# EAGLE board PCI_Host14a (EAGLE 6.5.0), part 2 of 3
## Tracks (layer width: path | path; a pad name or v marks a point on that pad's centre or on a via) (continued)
IDSEL2  (via drill 0.2, 0.3) (continued)
  Top 0.254: IC1.91 44.39,56.75 41.77,54.13 24.62,54.13 | v12.4,63.58 12.42,63.6 14.95,63.6 15.49,63.06 v15.88,63.06 15.8,63.06
  Top 0.305: v15.87,54.76 15.89,54.74 15.89,54.25 v17.05,53.09 | v20.35,49.96 v21.94,49.96 | v24.56,54.08 24.62,54.13
  Bottom 0.152: X1.J3-D18 6.1,64.21 11.76,64.21 v12.4,63.58
  Bottom 0.254: v12.4,63.58
  Bottom 0.305: 15.87,54.74 v15.88,63.06 | 15.87,54.74 15.87,54.6 | v17.05,53.09 17.05,50.44 17.53,49.96 v20.35,49.96 | v21.94,49.96 21.94,50.97 22.72,51.75 23.51,51.75 24.78,53.02 24.78,53.86 v24.56,54.08 | v15.87,54.76 15.87,54.74
IDSEL3  (via drill 0.2, 0.3)
  Top 0.152: v52.56,26.04 52.56,26.99 51.93,27.62 51.93,33.81 49.23,36.51 49.23,39.69 v48.91,40 | 45.57,45.24 45.56,45.23 v45.26,45.23 | 1.28,20.48 1.28,22.38
  Top 0.254: v47.96,45.24 45.57,45.24 | v44.78,47.15 44.78,47.62 v43.83,48.58 | IC1.90 44.1,57.26 41.76,54.92 v41.45,54.92 | v1.44,59.69 1.44,41.12 2.08,40.48 2.08,25.08 1.6,24.61 1.6,23.65 1.44,23.49 | 1.44,23.49 | 1.44,23.49 1.28,23.34 1.28,22.38 | 1.28,20.48 1.28,20 1.6,19.68 1.6,19.21 1.76,19.05 1.76,18.57 2.68,17.65
  Top 0.305: v17.54,25.2 17.54,18.34 16.93,17.73 v15.71,17.73 | v2.76,17.73 2.68,17.65
  Bottom 0.152: v43.83,48.58 43.83,48.89 | v45.26,45.23 45.26,46.67
  Bottom 0.254: 1.57,65.21 X1.J3-D19 | 1.57,65.21 | v41.45,54.92 41.45,51.28 43.83,48.89 | v48.91,40 48.91,44.13 v47.96,45.24 | 45.26,46.67 v44.78,47.15 | 1.57,65.21 | 1.57,65.21 1.28,64.93 1.28,59.85 v1.44,59.69
  Bottom 0.305: v17.54,25.2 18.76,26.42 52.14,26.42 52.44,26.11 v52.56,26.04 | v2.76,17.73 v15.71,17.73
INTA#  (via drill 0.2, 0.3)
  Top 0.152: 9.18,85.21 10.33,86.2 v12.71,86.2 | 64.17,80.06 64.17,71.37 64.33,71.22 64.33,70.61 64.48,70.46 64.48,70 64.94,69.53 64.94,67.76 v63.98,66.8 | v59.45,63.3 v59.45,59.59 | v64.31,56.61 v70.82,56.61 | IC1.47 64.05,62.76 64.2,62.9 v64.75,63.44
  Top 0.254: X1.J3-B29 9.18,85.21 | v15.33,86.12 17.87,86.12 18.75,85.25 22.4,85.25
  Top 0.305: v73.93,57.2 73.93,55.07 73.78,54.92 73.78,39.52 74.54,39.52 74.69,39.37 74.69,37.69 R2.2 | v25.77,92.41 25.77,86.46 23.94,86.46 23.79,86.31 23.64,86.31 23.48,86.16 23.48,86 23.33,85.85 23.33,85.24 22.42,85.24 22.4,85.25 | v62.35,98.35 62.35,99.42 62.5,99.57 63.87,99.57 63.87,98.5 63.72,98.35 63.72,88.9 63.87,88.75 64.33,88.75 64.33,85.85 64.17,85.7 64.17,84.02 64.33,83.87 64.33,80.21 64.17,80.06 | v25.41,93.98 v25.41,95.73 | v25.41,98.9 28.72,98.9 28.95,99.12 v29.3,99.12
  Bottom 0.152: v59.45,59.59 59.51,59.53 60.82,59.53 63.52,56.83 63.52,56.77 63.71,56.57 64.27,56.57 v64.31,56.61 | 59.76,66.95 63.83,66.95 v63.98,66.8 | 73.88,57.15 71.35,57.15 v70.82,56.61 | v59.45,63.3 63.79,63.3 64.15,63.66 64.53,63.66 v64.75,63.44
  Bottom 0.254: v12.71,86.2 15.02,86.2 v15.33,86.12
  Bottom 0.305: v62.35,98.35 62.19,98.2 34.06,98.2 33.19,99.06 29.36,99.06 v29.3,99.12 | 59.76,66.95 59.6,66.8 59.6,64.52 59.45,64.36 v59.45,63.3 | 73.88,57.15 v73.93,57.2 | v25.77,92.41 25.77,93.62 v25.41,93.98 | v25.41,95.73 v25.41,98.9 | 63.52,56.83
INTB#  (via drill 0.2, 0.3)
  Top 0.152: 7.12,85.21 v8.03,84.3 | 66.16,83.57 66.16,80.52 | IC1.48 63.44,63.26 63.99,63.82 64.47,64.29 | 64.47,64.29 | 64.47,64.29 64.63,64.45 64.63,64.93 v64.65,64.93 65,65.31 65,65.46 65.1,65.56 | 66.31,80.37 66.31,66.79 65.8,66.28 65.8,66.26 65.1,65.56 | 65.1,65.56 | 78.5,61.47 78.5,64.78 v78.35,64.94
  Top 0.254: X1.J3-C29 7.12,85.21 | 22.72,82.87 18.91,82.87 17.8,83.98 17.32,83.98 16.29,85.01 v14.46,85.01
  Top 0.305: v72.41,53.7 72.56,53.54 72.56,39.37 72.25,39.37 72.1,39.22 72.1,37.69 R2.3 | v78.2,53.7 78.35,53.85 78.35,59.49 78.2,59.64 78.2,61.32 78.35,61.47 78.5,61.47 | v23.18,82.35 23.18,82.8 22.72,82.8 22.72,82.87 | v27.6,82.35 31.41,82.35 v31.41,79.91 | v39.64,79.91 39.49,80.06 39.49,83.72 v39.64,83.87 | v66.31,83.72 66.16,83.57 | 66.16,80.52 66.31,80.37
  Bottom 0.152: 13.75,84.3 13.67,84.22 8.11,84.22 v8.03,84.3 | v78.35,64.94 64.82,64.94 v64.65,64.93
  Bottom 0.254: 13.75,84.3 v14.46,85.01
  Bottom 0.305: v72.41,53.7 72.56,53.54 78.04,53.54 v78.2,53.7 | v23.18,82.35 v27.6,82.35 | v31.41,79.91 v39.64,79.91 | v39.64,83.87 39.79,84.02 64.94,84.02 65.09,83.87 65.09,83.72 v66.31,83.72
INTC#  (via drill 0.2, 0.3)
  Top 0.152: 4.3,88.58 13.99,88.58 | v65.55,84.48 65.55,80.37 | 65.7,80.21 65.7,67.27 v64.94,66.52 64.57,66.14 64.41,66.14 63.99,65.72 63.99,64.51 63.24,63.76 IC1.49
  Top 0.254: v4.14,88.42 | v4.14,88.42 4.3,88.58 | 13.99,88.58 v14.62,87.95 | v17.32,85.25 | v17.32,85.25 17.8,84.77 18.11,84.77 18.59,84.3 | 18.59,84.3 | 18.59,84.3 18.75,84.14 21.92,84.14
  Top 0.305: v69.51,43.03 69.51,37.69 R2.4 | v75.15,43.03 75.3,43.18 75.3,48.36 75.15,48.51 75.15,57.51 v75,57.66 | v85.36,57.81 85.21,57.96 85.21,66.04 v85.36,66.19 | 26.23,84.78 26.23,85.85 24.09,85.85 23.94,85.7 23.94,84.18 21.96,84.18 21.92,84.14 | 26.23,84.78 26.07,84.63 | v32.17,82.42 32.17,77.01 31.68,76.52 28.59,76.52 28.11,76.99 | 65.55,80.37 65.7,80.21 | 26.23,84.78 26.22,84.78 26.05,84.61 26.05,78.74 25.73,78.42 25.73,78.11 26.21,77.63 27.48,77.63 28.11,76.99 | 28.11,76.99 | v38.12,84.78 38.12,82.89 v37.64,82.42
  Bottom 0.152: 5.09,85.41 3.98,86.52 3.98,88.27 | 79.87,66.95 79.85,66.93 67.26,66.93 66.85,66.52 v64.94,66.52
  Bottom 0.254: X1.J3-D29 5.09,85.41 | 3.98,88.27 v4.14,88.42 | v14.62,87.95 14.46,88.11 17.16,85.41 | 17.16,85.41 | 17.16,85.41 v17.32,85.25
  Bottom 0.305: v69.51,43.03 69.66,43.18 75,43.18 v75.15,43.03 | v75,57.66 75.15,57.81 75.3,57.81 75.45,57.96 85.21,57.96 v85.36,57.81 | v85.36,66.19 80.94,66.19 80.79,66.34 80.79,66.95 79.87,66.95 | v38.12,84.78 38.12,84.48 39.18,84.48 39.33,84.63 65.39,84.63 v65.55,84.48 | v32.17,82.42 v37.64,82.42
INTD#  (via drill 0.2)
  Top 0.152: X1.J3-B28 9.33,83.21 10.33,84.22 15.81,84.22 | v74.54,79.15 73.17,79.15 v73.17,80.67 | v63.57,80.52 63.57,71.22 63.72,71.07 63.72,70.46 63.87,70.31 63.87,69.55 64.02,69.39 64.17,69.39 64.17,68.61 63.36,67.79 63.36,64.93 63.04,64.61 62.5,64.61 IC1.50
  Top 0.254: 15.81,84.22 15.93,84.09
  Top 0.305: v67.38,43.79 67.53,43.64 67.53,39.52 67.22,39.52 67.07,39.37 67.07,37.69 R2.5 | v96.03,47.3 v96.03,43.79 | v92.22,54.92 92.06,55.07 92.06,58.11 92.22,58.27 92.22,59.18 92.06,59.33 91.15,59.33 91.15,61.92 91,62.08 91,62.38 90.84,62.53 89.02,62.53 89.02,70.92 v89.17,71.07 | v16.02,84.33 16.02,84.18 15.93,84.09 | v18.76,91.19 18.46,91.19 18.46,91.49 18.3,91.64 18.15,91.64 v18.15,95.3 | v54.42,113.59 54.42,112.52 54.57,112.37 54.57,111.76 54.42,111.61 54.42,110.08 54.57,109.93 54.57,109.17 54.73,109.02 54.88,109.02 54.88,104.75 55.03,104.6 57.62,104.6 57.62,97.89 57.47,97.74 57.47,88.44 57.62,88.29 58.23,88.29 58.23,80.82 v58.08,80.67 | v11.45,98.2 12.94,98.2 13.19,97.95 13.19,95.3 v13.35,95.14
  Bottom 0.152: 66.16,80.82 71.95,80.82 | 63.72,80.67 66,80.67 | v58.08,80.67 63.57,80.67
  Bottom 0.305: v67.38,43.79 78.35,43.79 78.5,43.94 78.5,44.09 89.47,44.09 89.63,43.94 89.63,43.79 v96.03,43.79 | v96.03,47.3 96.03,47.6 95.72,47.6 95.57,47.75 95.57,50.19 95.72,50.34 95.88,50.34 96.03,50.5 96.03,51.56 98.62,51.56 98.77,51.71 98.77,53.24 98.92,53.39 98.92,54.76 97.25,54.76 97.09,54.92 v92.22,54.92 | v89.17,71.07 89.02,71.22 85.21,71.22 85.05,71.07 84.14,71.07 83.99,71.22 83.99,79.15 v74.54,79.15 | v73.17,80.67 72.1,80.67 71.95,80.82 | 66,80.67 66.16,80.82 | 63.72,80.67 v63.57,80.52 63.57,80.67 | v16.02,84.33 16.17,84.48 17.85,84.48 18,84.63 18,84.78 18.15,84.94 18.15,86.31 17.54,86.31 17.39,86.46 17.39,89.05 17.54,89.2 18.76,89.2 18.91,89.36 18.91,91.19 v18.76,91.19 | v11.45,98.2 11.29,98.35 11.29,106.84 12.09,107.64 18.3,107.64 19.07,108.41 19.07,112.94 19.87,113.74 54.27,113.74 v54.42,113.59 | v18.15,95.3 13.51,95.3 v13.35,95.14
IRDY#  (via drill 0.2, 0.3)
  Top 0.152: IC1.55 58.15,65.33 58.32,65.17 60.86,65.17 v60.98,65.28 | X1.J3-C13 7.03,53.21 6.05,52.23 5.69,52.23 5.67,52.21 4.42,52.21 4.38,52.17 4.16,52.17 v4.14,52.19 | v7.04,25.06 12.7,25.06
  Top 0.254: 12.7,25.06 12.89,25.06 v13.51,24.45
  Top 0.305: v13.51,29.53 21.92,29.53 22.72,30.32 37.16,30.32 37.2,30.38 v37.2,28.09 | v77.74,64.21 77.74,59.33 77.89,59.18 77.89,54.3 77.59,54 v77.59,52.93 | v74.39,52.93 74.23,52.78 74.23,40.59 75.15,39.67 75.15,39.22 75.61,38.76 75.61,35.56 74.23,34.19 74.23,32.21 73.32,31.29 v73.32,30.53 | v76.83,30.23 76.83,29.31 76.98,29.16 v76.98,17.27 | v55.64,16.66 55.64,17.42 55.49,17.58 v55.49,20.17 | v43.45,20.32 43.6,20.47 43.6,27.94 v43.45,28.09
  Bottom 0.152: 82.16,65.13 80.94,65.13 80.94,64.68 80.47,64.21 v77.74,64.21 67.8,64.21 | v4.14,52.19 3.21,52.19 2.69,51.67 2.69,50.76 2.34,50.4 2.16,50.4 1.92,50.17 1.92,41.12 2.71,40.32 2.71,38.38 2.91,38.18 2.91,27.58 3.35,27.15 3.51,27.15 4.62,26.04 6.07,26.04 v7.04,25.06 | v13.51,24.45 v13.51,29.53
  Bottom 0.305: v60.98,65.28 60.98,64.21 67.8,64.21 68.29,64.21 | 82.16,65.13 R1.3 | v77.59,52.93 77.43,53.09 74.54,53.09 v74.39,52.93 | v73.32,30.53 73.62,30.23 v76.83,30.23 | v76.98,17.27 76.83,17.42 62.19,17.42 62.04,17.27 61.13,17.27 60.52,16.66 v55.64,16.66 | v55.49,20.17 55.34,20.02 44.67,20.02 44.36,20.32 v43.45,20.32 | v43.45,28.09 43.3,27.94 37.35,27.94 v37.2,28.09
LED_A  (via drill 0.2, 0.3)
  Top 0.152: v63.41,68.94 63.26,69.09 63.26,70.16 63.11,70.31 63.11,70.92 62.96,71.07 62.96,80.06 | 46.19,64.36 46.19,65.27 45.89,65.56 45.89,67.41 v46.03,67.55 | v74.15,98.42 74.15,99.7
  Top 0.305: 62.96,80.06 62.8,80.21 62.65,80.21 62.65,86.16 62.8,86.31 62.96,86.31 62.96,88.75 63.11,88.9 v63.11,98.81 | 74.15,99.7 R5.1 | IC1.76 46.19,64.36
  Bottom 0.152: 71.71,98.96 73.62,98.96 v74.15,98.42 | v63.41,68.94 63.29,69.22 61.29,69.22 60.98,68.9 59.86,68.9 59.07,69.69 57.64,69.69 57.32,70.01 51.77,70.01 51.13,69.37 51.13,67.63 50.66,67.15 46.53,67.15 46.13,67.55 v46.03,67.55
  Bottom 0.254: 71.61,98.96 71.71,98.96
  Bottom 0.305: v63.11,98.81 63.26,98.96 71.61,98.96
LED_B  (via drill 0.2)
  Top 0.152: v71.76,77.76 71.76,69.42 v72.08,69.1
  Top 0.305: v91,67.41 91,66.34 90.84,66.19 90.24,66.19 90.24,65.13 LED2.C | v46.95,68.17 46.95,67.72 47.26,67.72 47.41,67.56 47.41,66.34 48.02,66.34 IC1.75 | v47.56,74.57 v47.56,78.38
  Bottom 0.152: 71.03,78.23 71.03,78.21 71.29,77.95 71.58,77.95 v71.76,77.76 | v72.08,69.1 72.08,69.06 72.56,68.58 80.43,68.58 80.79,69.09
  Bottom 0.305: 80.79,69.09 84.29,69.09 84.45,68.94 84.45,67.56 89.78,67.56 89.93,67.72 90.84,67.72 91,67.56 v91,67.41 | v46.95,68.17 46.95,69.09 46.8,69.24 46.65,69.24 46.65,73.36 46.5,73.36 46.34,73.51 46.34,74.57 v47.56,74.57 | v47.56,78.38 47.72,78.23 57.77,78.23 57.93,78.38 70.88,78.38 71.03,78.23
LOCK#  (via drill 0.2, 0.3)
  Top 0.152: 12.71,50.64 14.86,50.64 17.16,48.34 17.32,48.34 18.35,47.31 | 18.35,47.31 | 18.35,47.31 18.43,47.23 24.14,47.23 24.22,47.15 26.53,47.15 v27,47.62 | v27,47.62
  Top 0.305: v12.56,50.64 12.66,50.65 12.71,50.64 | v40.18,87.95 40.34,87.79 40.34,83.33 v40.4,83.26 40.5,83.17 40.5,79.38 39.23,78.11 35.89,78.11 v31.29,73.5
  Bottom 0.152: 7.95,50.17 12.08,50.17 | 72.73,82.22 73.83,81.12 73.83,77.15 73.99,76.99 73.99,74.93 75.1,73.82 75.1,72.87 75.26,72.71 R1.6 | 58.69,81.89 65.7,81.89 65.85,82.04 71.95,82.04 | 31.29,72.39 29.86,70.96 29.86,68.74 29.54,68.42 29.54,57.47 27.96,55.88 27.96,48.58 v27,47.62
  Bottom 0.254: X1.J3-C11 7.09,49.31 7.95,50.17 | 12.08,50.17 v12.56,50.64
  Bottom 0.305: v40.4,83.26 40.55,83.41 55.03,83.41 55.18,83.26 55.18,82.04 58.54,82.04 58.69,81.89 | 71.95,82.04 72.1,82.19 72.71,82.19 72.73,82.22 | 39.54,88.27 v30.81,88.27 | 39.54,88.27 | 39.54,88.27 39.86,88.27 v40.18,87.95 | 31.29,72.39 v31.29,73.5
N$2  (via drill 0.2)
  Top 0.305: v92.22,93.93 92.22,88.14 92.37,87.99 92.37,70.46 92.06,70.46 91.91,70.31 91.91,70 91.76,69.85 91.76,67.26 92.83,67.26 92.98,67.11 92.98,65.13 LED2.A
  Bottom 0.254: 86.46,93.78 86.46,99.93
  Bottom 0.305: v92.22,93.93 92.06,93.78 86.46,93.78 | R5.2 85.11,101.28 86.46,99.93
N$3
  Top 0.305: J2.4 20.28,112.22 17.85,112.22 J2.2 | 37.05,112.22 35.68,112.22 J3.2 | 37.05,112.22 38.12,112.22 J3.4 | 37.05,112.22 37.05,108.1 36.44,108.1 36.29,107.95 36.29,103.23 JP3.1
  Bottom 0.305: J2.4 20.44,112.06 21.2,112.06 22.27,111 23.33,111 24.4,112.06 35.52,112.06 J3.2
N$4  (via drill 0.2)
  Top 0.152: 76.37,48.82 v76.37,102.31
  Top 0.305: v84.6,16.05 84.6,21.39 L1.2 | 66.08,14.45 66.16,14.38 66.92,14.38 66.92,12.7 C18.+ 66.92,12.55 | 66.08,14.45 66,14.53 66,18.34 IC3.4 | 73.47,19.86 69.36,19.86 69.2,20.02 69.2,25.65 IC3.20 | 76.37,48.82 76.52,48.67 76.52,39.22 76.37,39.06 76.06,39.06 76.06,34.04 75.91,33.88 74.69,33.88 74.69,29.16 74.84,29.01 74.84,21.84 74.69,21.69 73.47,21.69 73.47,19.86 | v66.16,14.83 66.16,14.53 66.08,14.45 | R9.2 70.88,3.56 70.88,7.52 R8.2 70.88,7.67 v70.88,14.83 | v73.47,15.75 73.47,19.86
  Bottom 0.305: v84.6,16.05 81.85,16.05 81.7,16.2 76.22,16.2 76.06,16.05 76.06,15.75 74.39,15.75 74.31,15.67 | 74.31,15.67 74.23,15.6 74.23,14.83 v70.88,14.83 v66.16,14.83 59.76,14.83 JP5.1 | v76.37,102.31 76.22,102.46 69.2,102.46 69.2,102.16 69.05,102.01 67.07,102.01 67.07,102.92 66.92,103.07 65.85,103.07 C17.1 | v73.47,15.75 74.23,15.75 74.31,15.67
N$5
  Top 0.305: LED3.A 83.53,4.01 82.31,4.01 82.31,5.38 82.16,5.54 81.79,5.54 81.3,6.03 81.3,7.3 R8.1
N$9
  Bottom 0.305: IC2.1 78.96,41.5 79.87,41.5 80.03,41.35 80.03,36.47 86.58,36.47 C11.1
N$10  (via drill 0.2)
  Top 0.305: 16.62,107.04 12.82,107.04 12.82,102.46 JP9.1 | 16.62,107.04 17.22,107.04 17.8,107.61 | v66.31,87.22 66.46,87.38 66.46,91.95 66.31,92.1 66.31,92.86 66.46,92.86 66.61,93.02 66.61,95.61 66.77,95.76 66.77,96.67 66.61,96.83 66.61,96.98 66.46,96.98 66.31,97.13 66.31,100.64 66.46,100.79 66.46,101.7 66.16,101.7 66,101.85 65.39,101.85 65.24,101.7 63.72,101.7 63.57,101.85 63.57,109.02 63.72,109.17 63.72,114.35 56.4,114.35 56.25,114.2 56.25,113.74 v56.1,113.59 56.1,113.62 55.42,114.3 53.2,114.3 53.04,114.14 16.84,114.14 15.73,113.03 15.73,110.81 16.69,109.85 16.62,109.78 16.62,107.04 | v105.32,86.77 105.48,86.61 105.48,64.36 104.87,63.75 104.71,63.75 104.71,63.6 104.56,63.45 104.56,61.62 104.71,61.47 104.87,61.47 104.87,48.36 v104.71,48.21 | v97.4,47.3 97.55,47.14 97.55,44.55 v97.4,44.4 | v77.89,44.55 77.74,44.4 77.74,39.22 77.89,39.06 78.5,39.06 78.5,36.17 78.35,36.02 77.74,36.02 77.74,32.21 77.59,32.05 77.43,32.05 77.43,31.29 77.59,31.14 77.59,29.31 77.43,29.16 77.43,21.84 77.59,21.69 78.81,21.69 78.81,21.39 78.96,21.23 78.96,20.78 79.11,20.62 79.11,20.02 78.96,19.86 v78.96,18.19 | X3.2 29.43,7.67 29.43,16.66 C26.+ 29.43,16.81 v29.43,19.56 | v15.71,21.84 16.93,20.62 v16.93,19.86
  Bottom 0.305: v105.32,86.77 94.2,86.77 94.05,86.61 82.77,86.61 82.77,87.38 82.62,87.53 75.16,87.53 74.79,87.15 72.88,87.15 72.72,87.31 66.4,87.31 v66.31,87.22 | v104.71,48.21 101.97,48.21 101.82,48.06 101.82,47.9 101.51,47.9 101.36,47.75 101.36,47.45 101.06,47.45 100.9,47.3 v97.4,47.3 | v97.4,44.4 97.25,44.55 94.81,44.55 94.66,44.4 89.93,44.4 89.63,44.7 78.04,44.7 v77.89,44.55 | v78.96,18.19 78.81,18.34 61.59,18.34 61.43,18.19 59.76,18.19 JP10.3 59.6,18.19 58.84,18.19 57.62,19.41 55.49,19.41 55.34,19.56 44.06,19.56 v44.06,19.71 43.91,19.56 39.49,19.56 39.33,19.41 32.93,19.41 32.78,19.56 30.95,19.56 30.8,19.41 29.43,19.41 v29.43,19.56 29.28,19.41 24.55,19.41 24.4,19.56 22.57,19.56 22.27,19.86 v16.93,19.86 | v15.71,21.84 14.34,21.84 JP11.1
N$11
  Top 0.305: C11.2 89.17,36.63 89.17,38.3 89.02,38.46 87.64,38.46 87.64,43.03 87.49,43.18 83.99,43.18 83.99,41.5 IC2.3
N$13
  Top 0.305: IC2.4 86.58,41.35 86.58,38 86.73,37.85 88.1,37.85 88.1,36.17 88.25,36.02 88.25,33.12 88.41,32.97 89.02,32.97 89.02,32.66 89.17,32.51 89.17,30.38 89.32,30.23 91.91,30.23 91.91,34.65 92.06,34.8 92.52,34.8 92.52,36.47 C12.1
N$14
  Top 0.305: J1.2 53.36,112.06 53.36,111.15 53.2,111 48.94,111 48.94,103.23 JP1.1
N$15  (via drill 0.2)
  Top 0.152: 75.76,99.26 75.76,76.1 75.61,75.95 74.84,75.95 74.84,70.46 75,70.31 75.76,70.31 75.76,48.67
  Top 0.305: v22.88,100.48 22.88,100.18 20.74,100.18 20.59,100.33 20.59,103.53 20.44,103.53 20.28,103.68 20.28,109.47 J2.3 | 75.76,99.26 v75.61,99.42 | 75.76,48.67 75.91,48.51 75.91,39.83 v75.76,39.67
  Bottom 0.305: v22.88,100.48 23.03,100.64 29.08,100.64 29.99,99.72 34.15,99.72 34.3,99.87 39.49,99.87 39.64,99.72 46.8,99.72 46.95,99.87 46.95,100.03 54.88,100.03 55.03,99.87 55.03,99.72 60.98,99.72 61.13,99.57 74.39,99.57 74.54,99.42 v75.61,99.42 | v75.76,39.67 75.76,34.19 70.27,34.19 70.12,34.04 59.3,34.04 59.15,34.19 59.15,34.34 58.08,34.34 57.93,34.19 57.93,33.43 56.71,33.43 56.55,33.27 56.4,33.27 56.25,33.12 56.25,32.97 54.42,32.97 54.27,32.82 54.27,31.29 53.2,31.29 JP2.8 53.05,31.29 52.14,31.29 52.14,30.38 51.98,30.23 51.22,30.23 51.07,30.07 50.16,30.07 50,30.23 49.55,30.23 49.39,30.38 49.09,30.38 49.09,31.14 48.94,31.29 48.17,31.29 JP2.4
N$16
  Top 0.305: C12.2 95.11,36.63 95.11,39.52 94.96,39.67 92.67,39.67 92.67,42.72 92.52,42.88 92.37,42.88 92.37,43.03 92.22,43.18 89.02,43.18 89.02,41.5 IC2.5
N$17  (via drill 0.2)
  Top 0.305: v81.09,32.51 80.94,32.66 80.94,39.98 81.09,40.13 81.4,40.13 81.4,41.35 IC2.2
  Bottom 0.305: v81.09,32.51 79.87,32.51 79.87,31.75 79.72,31.6 78.65,31.6 C13.2
N$18  (via drill 0.2)
  Top 0.305: v93.74,56.44 93.74,50.95 94.05,50.95 94.2,50.8 94.2,49.12 IC2.10
  Bottom 0.305: v93.74,56.44 89.47,56.44 JP4.2
N$19
  Bottom 0.305: IC2.9 96.79,49.12 99.38,49.12 99.53,49.28 99.53,49.58 100.9,49.58 101.06,49.73 101.06,50.19 101.21,50.19 101.36,50.34 101.36,50.5 101.67,50.5 101.82,50.65 101.82,54.15 104.71,54.15 104.87,54.3 104.87,55.83 105.32,55.83 105.48,55.98 105.48,61.47 98.01,61.47 97.86,61.32 97.86,60.25 97.25,60.25 97.09,60.1 93.13,60.1 92.98,59.94 92.98,57.81 91.15,57.81 91,57.96 88.56,57.96 88.41,57.81 88.41,57.2 88.25,57.05 88.25,55.98 88.41,55.83 88.41,54 89.32,54 JP4.4
N$21
  Top 0.305: C10.1 90.24,31.6 90.24,34.95 90.39,35.1 91.15,35.1 91.15,39.52 91.3,39.67 91.61,39.67 91.61,41.35 IC2.6
N$22  (via drill 0.2)
  Top 0.305: JP7.5 90.39,78.38 90.39,77.47 91.61,76.25 91.61,75.49 90.39,74.27 90.39,73.36 JP7.1 | v82.62,56.74 82.62,54.92 82.46,54.76 82.46,53.7 82.62,53.7 82.77,53.54 82.77,51.56 83.83,51.56 83.99,51.41 83.99,49.12 IC2.14 | v84.75,56.74 84.6,56.9 84.6,66.5 84.75,66.65 84.75,69.09 84.6,69.24 84.6,71.68 v84.75,71.83
  Bottom 0.305: v82.62,56.74 v84.75,56.74 | v84.75,71.83 89.17,71.83 89.32,71.98 89.32,73.36 90.24,73.36 JP7.1
N$23
  Top 0.305: 89.4,77.7 90.39,76.71 90.39,75.95 JP7.3 | 89.4,77.7 89.17,77.93 89.17,78.84 90.39,80.06 90.39,80.82 JP7.7 | IC2.13 86.58,49.12 86.58,52.32 86.73,52.48 87.8,52.48 87.8,52.78 87.95,52.93 87.95,53.39 88.1,53.54 88.1,54.3 87.95,54.46 87.95,55.98 88.1,56.13 88.1,57.05 88.25,57.2 88.41,57.2 88.41,72.29 88.56,72.44 88.86,72.44 88.86,72.75 89.02,72.9 89.02,73.81 89.17,73.97 89.32,73.97 89.32,77.62 89.4,77.7
N$24
  Top 0.305: JP7.8 87.8,80.82 87.8,80.06 86.58,78.84 86.58,75.49 87.8,74.27 87.8,73.36 JP7.2
  Bottom 0.305: J6.2 100.29,81.43 98.47,81.43 98.47,79.3 98.31,79.15 97.86,79.15 97.7,78.99 97.55,78.99 97.55,78.84 97.4,78.69 96.03,78.69 J4.3 95.88,78.69 92.06,78.69 91.91,78.84 91.91,79.3 91.61,79.3 91.45,79.45 91,79.45 90.84,79.6 89.93,79.6 89.78,79.76 89.78,79.91 89.02,79.91 88.86,80.06 88.86,80.98 87.95,80.98 JP7.8
N$26
  Top 0.305: JP7.6 87.8,78.38 87.8,75.95 JP7.4
  Bottom 0.305: J6.3 100.29,78.69 98.62,78.69 98.47,78.54 98.01,78.54 97.86,78.38 97.86,76.4 97.7,76.25 96.03,76.25 J4.2 95.88,76.25 94.2,76.25 94.2,76.71 94.05,76.86 91,76.86 90.84,77.01 89.78,77.01 89.63,76.86 89.32,76.86 89.17,76.71 88.86,76.71 88.86,76.1 88.71,75.95 87.95,75.95 JP7.4
N$27  (via drill 0.2)
  Top 0.305: IC2.7 94.2,41.5 v94.2,45.77 93.28,45.77 93.13,45.92 93.13,55.52 v92.98,55.68
  Bottom 0.305: v94.2,45.77 100.29,45.77 J7.3 | v92.98,55.68 94.35,55.68 94.35,55.98 94.5,56.13 95.88,56.13 J5.2
N$28  (via drill 0.2)
  Top 0.305: v98.92,41.5 98.77,41.66 98.77,47.14 98.85,47.22 | 98.85,47.22 98.92,47.3 100.29,47.3 100.29,48.36 J7.2 | J5.3 95.88,58.72 95.88,57.81 96.03,57.66 98.31,57.66 98.31,54.61 98.77,54.15 98.77,47.3 98.85,47.22
  Bottom 0.305: v98.92,41.5 96.79,41.5 IC2.8
N$33  (via drill 0.2)
  Top 0.305: v92.98,88.44 92.98,68.94 LED1.A
  Bottom 0.305: v92.98,88.44 84.29,88.44 R4.2
N$35  (via drill 0.2)
  Top 0.305: v71.64,28.55 71.8,28.4 71.8,25.81 IC3.16 | v87.03,28.55 87.03,25.96 C15.1 | v97.4,24.43 97.4,23.37 97.55,23.22 97.55,19.41 98.31,19.41 98.47,19.56 100.14,19.56 X2.D-
  Bottom 0.305: v71.64,28.55 71.8,28.4 73.32,28.4 73.47,28.24 80.03,28.24 80.18,28.4 86.88,28.4 v87.03,28.55 | v97.4,24.43 97.25,24.28 95.42,24.28 95.27,24.13 90.24,24.13 90.08,24.28 87.95,24.28 87.8,24.43 87.8,25.81 87.03,25.81 C15.1
N$36  (via drill 0.2)
  Top 0.305: 21.88,19.33 21.05,18.49 21.05,16.81 C27.+ 21.05,16.66 v21.05,7.67 | 21.88,19.33 21.96,19.41 21.96,22.15 JP8.1 | 21.88,19.33 v21.96,19.25
  Bottom 0.305: JP6.1 16.47,15.75 18.3,15.75 19.22,16.66 20.89,16.66 C27.+ | v21.96,19.25 22.11,19.1 24.09,19.1 24.25,18.95 31.11,18.95 31.26,19.1 32.48,19.1 32.63,18.95 39.64,18.95 39.79,19.1 55.03,19.1 55.95,18.19 57.01,18.19 JP10.1 | v21.05,7.67 24.25,7.67 X3.1
N$37  (via drill 0.2)
  Top 0.305: v71.19,21.69 71.19,25.65 IC3.17 | v93.28,21.54 93.28,25.65 C19.1
  Bottom 0.305: v71.19,21.69 82.62,21.69 82.77,21.54 82.77,21.39 83.53,21.39 83.83,21.69 89.02,21.69 89.17,21.54 90.08,21.54 90.24,21.69 93.13,21.69 v93.28,21.54
N$38  (via drill 0.2)
  Top 0.305: v65.85,46.38 65.85,27.79 67.68,27.79 67.83,27.63 67.83,26.72 67.98,26.57 67.98,25.81 IC3.22 | v90.54,46.38 90.54,51.26 90.69,51.41 90.84,51.41 90.84,58.11 90.69,58.27 89.93,58.27 89.93,60.86 LED4.C
  Bottom 0.305: v65.85,46.38 71.49,46.38 71.64,46.53 90.39,46.53 v90.54,46.38
N$39  (via drill 0.2)
  Top 0.305: v67.38,19.71 67.38,25.65 IC3.23 | v83.38,18.95 83.38,14.99 83.53,14.83 83.53,14.07 83.38,13.92 83.38,6.76 83.53,6.76 LED3.C
  Bottom 0.305: v67.38,19.71 67.38,18.95 v83.38,18.95
N$40  (via drill 0.2)
  Top 0.305: v85.66,12.24 86.27,12.24 86.43,12.39 86.43,13.16 86.58,13.31 86.58,21.39 L1.1 86.58,21.54 v86.58,23.67 | v98.16,23.67 98.16,21.08 98.31,20.93 98.47,20.93 98.47,20.78 98.92,20.32 X2.D+
  Bottom 0.305: v85.66,12.24 78.2,12.24 C14.2 | v98.16,23.67 95.57,23.67 95.42,23.52 90.08,23.52 89.93,23.67 87.64,23.67 87.49,23.52 86.73,23.52 v86.58,23.67
N$41  (via drill 0.2)
  Top 0.152: 80.48,11.59 80.48,11.94
  Top 0.305: v92.67,62.84 92.67,61.01 LED4.A | v106.54,62.84 106.7,62.69 106.7,46.38 106.54,46.23 106.24,46.23 105.78,45.77 105.78,45.16 106.24,44.7 107.31,44.7 107.31,27.18 107.15,27.03 v106.54,27.03 | v81.55,26.87 81.55,26.42 81.7,26.26 81.7,25.2 81.55,25.04 81.55,17.27 81.4,17.12 80.48,17.12 80.48,11.94 | v79.57,3.56 79.57,8.74 80.48,9.65 80.48,11.59 80.48,11.79
  Bottom 0.305: v106.54,62.84 v92.67,62.84 | v106.54,27.03 94.81,27.03 94.66,27.18 81.7,27.18 81.55,27.03 v81.55,26.87 | v79.57,3.56 80.94,3.56 R9.1
N$46  (via drill 0.2)
  Top 0.305: v73.02,24.43 73.02,24.59 72.71,24.59 72.56,24.74 72.56,25.65 IC3.15 | v96.79,22.15 96.94,22 96.94,18.8 100.14,18.8 X2.VBUS | v83.22,22.15 83.22,25.65 C16.2
  Bottom 0.305: v73.02,24.43 75,24.43 75.15,24.28 82.16,24.28 82.31,24.43 82.31,25.65 83.07,25.65 C16.2 | v96.79,22.15 95.57,22.15 95.42,22.3 90.08,22.3 89.93,22.15 89.32,22.15 89.17,22.3 83.38,22.3 v83.22,22.15
N$101  (via drill 0.2)
  Top 0.305: v18.3,106.12 18.3,108.1 18,108.1 17.85,108.26 17.85,109.47 J2.1 | v69.36,106.73 69.51,106.58 69.51,94.54 v69.36,94.39 | v82.92,94.39 82.92,85.7 83.07,85.55 83.53,85.55 v83.53,85.39 | v104.26,85.24 104.41,85.09 104.41,69.55 v104.26,69.39 | v99.38,64.06 99.23,63.91 99.23,60.55 v99.38,60.4 | v103.65,55.07 103.8,54.92 103.8,51.11 v103.65,50.95 | v96.79,46.69 96.79,43.94 96.94,43.79 97.7,43.79 97.7,36.32 97.86,36.17 97.86,29.92 v97.7,29.77 | v54.27,30.23 54.27,31.75 54.12,31.9 54.12,32.05 53.97,32.21 53.81,32.21 53.66,32.36 53.2,32.36 53.05,32.51 53.05,32.66 v52.74,32.66
  Bottom 0.305: 48.55,32.44 48.48,32.51 47.72,32.51 47.56,32.36 47.11,32.36 46.95,32.21 46.65,32.21 46.65,31.45 46.5,31.29 45.58,31.29 JP2.2 | 48.55,32.44 48.63,32.36 49.39,32.36 49.55,32.21 49.55,31.45 49.7,31.29 50.61,31.29 JP2.6 | J2.1 17.69,109.47 | v18.3,106.12 18.46,105.97 28.82,105.97 28.97,106.12 30.8,106.12 30.95,106.27 52.59,106.27 52.74,106.43 52.74,106.58 52.9,106.58 53.05,106.73 53.81,106.73 53.97,106.88 69.2,106.88 v69.36,106.73 | v82.92,94.39 v69.36,94.39 | v83.53,85.39 83.68,85.55 94.5,85.55 94.66,85.7 104.1,85.7 104.26,85.55 v104.26,85.24 | v104.26,69.39 100.45,69.39 100.29,69.24 100.29,68.94 98.92,68.94 98.77,68.78 98.77,64.06 v99.38,64.06 | v99.38,60.4 99.38,60.1 99.08,60.1 98.92,59.94 98.92,59.64 98.77,59.49 98.77,56.74 98.92,56.59 99.08,56.59 99.23,56.44 99.23,56.29 99.38,56.13 99.53,56.13 99.69,55.98 99.69,55.83 99.84,55.68 99.84,55.07 v103.65,55.07 | v103.65,50.95 103.8,50.8 105.17,50.8 105.32,50.65 105.32,45.92 102.43,45.92 102.28,46.08 101.51,46.08 101.36,46.23 101.36,46.69 100.9,46.69 100.75,46.84 97.86,46.84 97.7,46.69 v96.79,46.69 | v97.7,29.77 86.43,29.77 86.27,29.62 86.12,29.62 85.97,29.46 78.65,29.46 78.5,29.62 76.52,29.62 76.37,29.77 63.87,29.77 63.72,29.92 62.96,29.92 62.8,30.07 62.8,30.23 62.5,30.23 62.35,30.38 62.35,30.68 62.19,30.84 62.19,31.6 62.04,31.75 61.89,31.75 61.74,31.9 61.74,32.21 61.43,32.21 61.28,32.36 57.77,32.36 57.62,32.21 57.47,32.21 57.32,32.05 57.32,31.9 57.16,31.75 57.16,30.99 57.01,30.84 56.86,30.84 56.71,30.68 56.71,30.23 56.25,30.23 56.1,30.07 55.34,30.07 55.18,30.23 v54.27,30.23
  Bottom 0.305: v52.74,32.66 52.59,32.82 48.78,32.82 48.63,32.66 48.63,32.51 48.55,32.44
PAR  (via drill 0.3)
  Top 0.152: 2.79,74.06 2.79,81.2 3.35,81.76 | X1.J3-D9 3.86,45.21 2.56,46.51 2.56,50.96 2.71,51.12 2.71,61.44 | 56.53,74.79 56.53,72.07 56.69,71.91 56.69,70.64 57.01,70.33 57.01,68.1 56.69,67.79 | 56.69,67.79 | 56.69,67.79 56.65,67.75 IC1.58 | 3.35,81.76 | 31.61,95.09
  Top 0.254: 2.71,73.98 2.79,74.06 | 2.71,73.98 | 2.71,73.98 2.48,73.74 2.48,71.83 2.79,71.52 2.79,67.07 3.19,66.67 3.19,64.37 3.83,63.74 3.83,63.02 3.35,62.55 3.35,62.07 2.71,61.44 | 3.35,81.76 3.35,89.06 | v15.41,94.3 15.26,94.14
  Top 0.305: 3.35,89.06 3.67,89.38 3.83,89.38 3.98,89.53 v3.98,89.69 4.84,90.55 10.2,90.55 10.41,90.77 12.04,90.77 12.28,91 12.28,93.48 13.11,94.32 15.39,94.32 v15.41,94.3 15.41,95.57 17,97.16 17.64,97.16 17.8,97.31 29.38,97.31 31.61,95.09 32.08,94.62 39.54,94.62 40.34,95.41 54.71,95.41 55.03,95.09 55.03,88.14 54.88,87.99 54.88,86.77 55.64,86.77 55.79,86.61 55.79,86.31 56.55,86.31 56.71,86.16 56.71,74.97 56.53,74.79
PERR#  (via drill 0.2, 0.3)
  Top 0.152: X1.J3-B10 9.6,47.21 10.49,48.1 | 10.49,48.1 10.57,48.18 12,48.18 12.71,47.47 | 10.49,48.1 | v74.54,77.78 73.02,77.78 73.02,74.88 | 12.71,47.47 | 12.71,47.47 12.79,47.39 15.18,47.39 16.37,46.2 16.84,46.2 16.92,46.2 17.56,45.56 29.07,45.56 29.23,45.72 29.7,45.72 v29.78,45.8 | IC1.43 67.6,60.76 68.44,61.59 68.44,63.5 67.33,64.61 67.33,64.93 68.59,66.2 68.59,70.48 69.23,71.12 69.23,74.31 v69.35,74.43
  Top 0.305: v73.17,74.73 73.02,74.88 | v41.3,75.15 39.96,75.15 39.54,75.56 37.64,75.56 37.32,75.25 v34.94,75.25
  Bottom 0.152: v29.78,45.8 29.78,47.39 29.86,47.47 | 29.86,47.47 | 29.86,47.47 30.02,47.62 30.02,54.93 31.45,56.36 | 31.45,60.64 32.88,62.07 32.88,64.29 33.35,64.77 | 58.08,75.95 68.69,75.95 69.07,75.56 69.07,74.7 v69.35,74.43 69.36,74.43 69.71,74.77 73.12,74.77 v73.17,74.73
  Bottom 0.305: v74.54,77.78 82.16,77.78 R1.8 | 58.08,75.95 57.93,76.1 42.24,76.1 v41.3,75.15 | 31.45,56.36 31.45,60.64 | v34.94,75.25 33.35,73.66 33.35,64.77
PME#  (via drill 0.3)
  Top 0.152: X1.J3-D10 5.47,47.21 6.44,48.18 7.56,48.18 8.11,48.74 8.11,51.75 8.59,52.23 12.4,52.23 12.71,51.91 13.51,51.91 13.83,52.23 14.54,52.23 16.76,50.01 16.76,49.53 | 16.76,49.53 | 16.76,49.53 17.32,48.97 | 17.32,48.97 | 17.32,48.97 17.4,48.89 17.72,48.89 18.83,47.78 24.3,47.78 24.46,47.62 25.97,47.62 27.72,49.37 v40.34,49.37 | 45.26,49.37 45.42,49.37 46.21,50.17 | 46.21,50.17 | 46.21,50.17 46.37,50.32 48.09,50.32 IC1.1
  Top 0.254: v40.34,49.37 45.26,49.37 | 8.59,52.23
PSON#  (via drill 0.3)
  Top 0.152: X1.J3-C9 6.88,45.21 5.89,46.2 4.46,46.2 3.83,46.83 3.51,46.83 v3.35,46.99 | v3.35,41.59 3.35,35.08 v3.51,34.92
  Top 0.254: v5.95,27.23 14.7,27.23 v14.78,27.3 | v14.94,24.61 16.21,24.61 v16.53,24.29 | v40.66,24.45 40.66,21.43 41.61,20.48 41.92,20.48 42.24,20.16 42.24,13.97 v42.56,13.65
  Bottom 0.152: v3.35,46.99 3.35,46.83 2.87,46.36 2.87,43.97 3.35,43.5 v3.35,41.59 | v3.51,34.92 3.51,31.91 3.83,31.59 3.83,28.26
  Bottom 0.254: 3.83,28.26 | 3.83,28.26 4.94,27.15 5.87,27.15 v5.95,27.23 | v14.78,27.3 14.78,24.77 v14.94,24.61 | v16.53,24.29 24.62,24.29 24.78,24.45 31.61,24.45 31.92,24.13 37.32,24.13 37.8,24.61 40.5,24.61 v40.66,24.45 | v42.56,13.65 47.8,13.65 48.12,13.33 48.12,9.21 X3.6
REQ0#  (via drill 0.2, 0.3)
  Top 0.152: IC1.6 50.65,51.6 50.96,51.91 v50.97,51.91 | v50.81,54.13 50.81,54.77 49.39,56.2 49.39,57.78 v49.55,57.94 | 25.1,57.15 v42.24,57.15 | 25.1,57.15 | v23.83,57.31 23.99,57.15 25.1,57.15
  Top 0.305: v14.34,81.13 14.49,80.98 16.78,80.98 16.93,80.82 20.28,80.82 v20.28,79.6 | v21.96,78.84 22.11,78.99 24.09,78.99 24.09,74.42 23.94,74.27 23.94,73.51 24.09,73.36 25.16,73.36 25.16,71.83 25.01,71.68 25.01,68.78 v25.16,68.63
  Bottom 0.152: v49.55,57.94 43.04,57.94 v42.24,57.15 | 23.83,67.31 23.83,67.26 v23.83,57.31 | v50.81,54.13 50.97,53.97 v50.97,51.91
  Bottom 0.305: v14.34,81.13 14.34,73.36 14.19,73.2 11.14,73.2 X1.J3-A23 | v20.28,79.6 20.28,78.84 v21.96,78.84 | v25.16,68.63 25.16,68.33 24.86,68.33 24.7,68.17 24.7,67.26 23.83,67.26 23.79,67.26
REQ1#  (via drill 0.2)
  Top 0.152: X1.J3-C23 7.09,73.28 7.95,74.14 | 8.03,74.22 18.3,74.22 18.35,74.22 | IC1.7 51.15,46.53 50.89,46.28 | v23.03,66.38 23,66.34 | 41.16,46.65 41.54,46.28
  Top 0.254: 7.95,74.14 | 7.95,74.14 8.03,74.22 | 41.54,46.28 50.89,46.28 | v24.24,54.92 40.27,54.92
  Top 0.305: v41.16,48.51 41.16,46.65 | 40.27,54.92 v40.43,54.77 | 18.3,74.27 18.3,74.22 18.3,74.12 18.43,74.14 18.46,74.12 18.61,74.12 18.76,73.97 18.76,73.51 18.91,73.36 18.91,73.2 19.07,73.05 19.22,73.05 19.37,72.9 19.37,72.75 19.52,72.59 19.68,72.59 19.83,72.44 19.83,72.29 19.98,72.14 20.13,72.14 20.28,71.98 20.28,71.83 20.44,71.68 21.81,71.68 v21.81,68.94 | v21.81,66.19 23.03,66.19 v23.03,66.38
  Bottom 0.152: v24.23,54.93 v24.24,54.92
  Bottom 0.254: 23.03,55.4 23.04,55.4 23.51,54.93 v24.23,54.93 | 40.43,50.83 40.43,50.78 41.16,50.04
  Bottom 0.305: v23.03,66.38 23.03,55.4 | v40.43,54.77 40.43,50.83 | 41.16,50.04 v41.16,48.51 | v21.81,68.94 v21.81,66.19
REQ2#  (via drill 0.2)
  Top 0.152: X1.J3-B24 10.1,76.2 11.76,76.2 12.08,75.88 13.67,75.88 | IC1.8 51.65,46.24 51.29,45.87 40.19,45.87 39.7,46.36 39.7,47.81 v39.79,47.9 | 42.4,65.09 42.4,64.97 v41.65,64.21
  Top 0.254: X1.J3-B24 | 13.67,75.88 16.68,75.88 16.84,76.04 | 16.84,76.04 | 16.84,76.04 17,76.2 17.95,76.2 18.75,75.41 19.22,75.41 19.38,75.41
  Top 0.305: v47.88,61 v47.88,54.66 | 42.4,65.09 42.4,66.83 41.92,67.31 40.66,67.31 39.99,66.65 31.41,66.65 31.4,66.66 26.07,66.66 25.89,66.83 25.57,66.83 24.55,67.86 v24.55,72.14 24.55,72.44 | v23.03,72.14 21.35,72.14 21.2,72.29 21.2,72.59 20.28,72.59 20.28,72.75 19.98,73.05 19.98,73.66 19.37,73.66 19.22,73.81 19.22,75.41
  Bottom 0.152: v47.88,54.66 47.48,54.26 47.48,51.44 45.58,49.53 45.58,49.13 44.07,47.62 40.07,47.62 v39.79,47.9 | v41.65,64.21 41.8,64.06 42.54,64.06
  Bottom 0.305: 42.54,64.06 42.69,63.91 42.69,63.3 45.43,63.3 45.58,63.14 45.73,63.14 45.89,62.99 45.89,62.84 46.04,62.69 46.19,62.69 46.34,62.53 46.34,62.38 46.5,62.23 46.65,62.23 46.8,62.08 46.8,61.92 46.95,61.77 47.11,61.77 47.26,61.62 47.26,61.47 47.41,61.32 47.41,61.16 v47.88,61 | v23.03,72.14 v24.55,72.14
REQ3#  (via drill 0.2, 0.3)
  Top 0.152: IC1.9 52.15,45.78 v51.68,45.31 | 78.65,69.55 78.65,69.85 78.5,70 78.5,72.14 78.2,72.44 78.2,79.6 | v48.8,54.66 48.75,54.7 48.75,60.96 v48.8,60.85 | v46.86,49.3 46.86,48.19 v47.49,47.55
  Top 0.254: v14.3,91.28 14.46,91.28 14.78,90.96 15.26,90.96 17.64,88.58 23.19,88.58 23.51,88.27 24.3,88.27
  Top 0.305: v78.96,60.86 79.11,61.01 79.11,69.39 78.96,69.55 78.65,69.55 | 78.2,79.6 78.5,79.91 78.5,84.78 78.65,84.94 78.65,85.85 78.5,86 77.59,86 77.59,94.76 v77.26,95.08 | v26.38,96.52 26.38,93.32 26.23,93.17 25.01,93.17 25.01,92.1 25.16,91.95 25.16,88.44 25.01,88.29 24.4,88.29 24.3,88.27 | v27.6,98.05 27.76,98.21 v29.14,98.21
  Bottom 0.152: 56.11,61.16 76.52,61.16 76.67,61.01 76.67,60.86 v78.96,60.86 | v51.68,45.31 51.61,45.24 49.55,45.24 47.49,47.3 v47.49,47.55 | 47.13,49.58 v46.86,49.3 48.33,50.77 48.33,53.87 | 76.22,97.79 73.04,97.79
  Bottom 0.254: 10.05,91.15 11.13,92.23 13.35,92.23 v14.3,91.28 | v48.8,54.66 48.8,54.34 48.33,53.87
  Bottom 0.305: v48.8,60.85 48.63,60.69 55.64,60.69 56.11,61.16 | v27.6,98.05 27.6,96.52 v26.38,96.52 | X1.J3-B30 9.1,89.05 10.04,89.99 10.04,91.14 10.05,91.15 | v29.14,98.21 29.19,98.27 32.72,98.27 33.4,97.59 56.4,97.59 56.55,97.43 57.16,97.43 57.32,97.59 72.84,97.59 73.04,97.79 | 76.22,97.79 76.85,97.16 76.85,95.49 v77.26,95.08
RES.
  Top 0.305: IC1.78 IC1.77
RESET#  (via drill 0.2, 0.3)
  Top 0.152: 57.96,61.75 v57.96,59.37 | 59.42,54.26 IC1.30 | v70.18,83.66 69.51,84.33 | v66.93,82.95 66.93,66.75 66.37,66.2 66.06,65.88 65.56,65.39 65.56,63.4 v65.72,63.24
  Top 0.254: v58.28,62.07 57.96,61.75 | 69.51,84.33 69.51,84.69
  Top 0.305: 69.97,96.22 69.97,92.56 69.86,92.46 69.86,89.7 69.51,89.34 69.51,84.69 | 69.97,96.22 v69.97,108.71 | v97.86,83.41 97.86,62.23 v97.7,62.08 | v105.93,43.33 106.08,43.18 106.08,28.55 105.93,28.4 103.65,28.4 103.65,23.22 103.8,23.06 104.1,23.06 104.1,17.73 103.95,17.58 103.65,17.58 v103.65,14.68 | v59.39,54.29 59.42,54.26 | v67.38,4.93 67.38,3.25 S1.3 | v78.96,4.93 79.11,5.08 v79.11,9.2 | 69.97,96.22 v70.12,96.22
  Bottom 0.152: v57.96,59.37 57.96,58.58 | v70.18,83.66 72,83.66 72.86,82.8 | v58.28,62.07 58.59,62.39 60.02,62.39 60.34,62.71 65.18,62.71 v65.72,63.24
  Bottom 0.254: v66.93,82.95 69.79,82.95 70.18,83.34 v70.18,83.66
  Bottom 0.305: v69.97,108.71 69.81,108.56 60.37,108.56 60.37,109.32 60.21,109.47 58.54,109.47 J1.5 | 72.86,82.8 85.82,82.8 85.97,82.96 85.97,83.57 95.42,83.57 95.57,83.41 v97.86,83.41 | v97.7,62.08 107.15,62.08 107.31,61.92 107.31,43.33 v105.93,43.33 | v103.65,14.68 103.65,13.92 94.5,13.92 94.35,14.07 94.35,14.22 92.37,14.22 92.22,14.07 89.32,14.07 89.17,14.22 86.58,14.22 86.43,14.07 86.43,9.96 84.6,9.96 84.45,10.11 80.79,10.11 80.64,9.96 80.64,9.2 79.42,9.2 79.34,9.27 | 79.34,9.27 79.26,9.35 79.26,9.5 | 57.96,58.58 58.28,58.58 59.39,57.47 v59.39,54.29 | v67.38,4.93 v78.96,4.93 | v79.11,9.2 79.26,9.2 79.34,9.27 | 70.12,96.2 C9.1 | 70.12,96.2 73.52,96.2 R3.1 | v70.12,96.22 70.12,96.2
RS232_RX  (via drill 0.2)
  Top 0.305: v82.92,33.58 82.92,43.79 88.86,43.79 89.02,43.94 89.02,48.97 IC2.12 | v58.69,33.58 58.54,33.43 58.54,32.36 58.38,32.21 58.38,32.05 58.23,31.9 58.23,31.29 JP2.12
  Bottom 0.305: v82.92,33.58 70.42,33.58 70.27,33.43 58.84,33.43 v58.69,33.58
RS232_TX  (via drill 0.2)
  Top 0.305: v71.19,47.14 71.34,46.99 71.34,40.59 71.19,40.44 70.73,40.44 v70.73,32.82
  Bottom 0.305: v71.19,47.14 90.54,47.14 90.54,48.97 90.69,49.12 91.61,49.12 IC2.11 | v70.73,32.82 56.86,32.82 56.71,32.66 56.71,31.29 55.79,31.29 JP2.10
RST#  (via drill 0.2)
  Top 0.152: IC1.29 68.7,53.76 68.75,53.82
  Top 0.305: v70.58,53.85 70.58,47.6 70.42,47.45 v70.42,45.01 | v106.54,45.47 107.31,45.47 107.31,100.64 107.15,100.79 v106.54,100.79 | v2.76,92.25 2.76,89.97 v2.91,89.82 | v68.75,53.85 68.75,53.82
  Bottom 0.152: v68.75,53.85 68.75,53.82 69.39,53.18 69.91,53.18 v70.58,53.85
  Bottom 0.305: v70.42,45.01 70.58,45.16 71.8,45.16 71.95,45.31 89.78,45.31 90.08,45.01 94.5,45.01 94.66,45.16 99.23,45.16 99.38,45.01 99.38,44.7 99.69,44.7 99.84,44.55 100.9,44.55 101.06,44.7 101.21,44.7 101.36,44.86 101.36,45.01 101.67,45.01 101.82,45.16 101.82,45.47 v106.54,45.47 | v106.54,100.79 106.54,101.7 86.58,101.7 86.43,101.85 86.43,103.84 81.24,103.84 81.09,103.68 71.8,103.68 71.64,103.84 71.64,107.34 53.66,107.34 53.51,107.19 52.74,107.19 52.59,107.04 52.44,107.04 52.29,106.88 52.29,106.73 30.65,106.73 30.5,106.58 28.67,106.58 28.51,106.43 21.2,106.43 21.05,106.58 21.05,106.73 17.54,106.73 17.39,106.88 17.39,107.04 14.19,107.04 14.04,106.88 14.04,97.43 10.84,97.43 10.68,97.59 10.68,99.11 3.52,99.11 3.37,98.96 3.37,98.65 1.69,98.65 1.54,98.5 1.54,96.83 1.39,96.67 1.39,93.78 1.54,93.62 1.54,92.25 v2.76,92.25 | v2.91,89.82 2.91,83.26 5.04,83.26 X1.J3-D28
RX0  (via drill 0.2, 0.3)
  Top 0.152: IC1.2 48.65,49.11 v48.35,48.82
  Top 0.305: JP2.3 48.17,28.7 50.61,28.7 JP2.5 | JP2.11 58.23,28.85 58.23,29.77 57.32,29.77 57.16,29.92 57.16,30.68 57.01,30.84 57.01,31.6 57.16,31.75 57.16,32.36 57.77,32.36 57.93,32.51 57.93,43.94 v57.87,43.9
  Bottom 0.152: v48.35,48.82 v48.36,48.82 53.11,48.82 54.78,47.15 54.78,45.24 56.37,43.66 57.63,43.66 v57.87,43.9
  Bottom 0.305: JP2.13 60.67,28.7 58.38,28.7 JP2.11 58.23,28.7 57.32,28.7 57.16,28.55 57.16,27.79 57.01,27.63 56.25,27.63 56.1,27.48 52.74,27.48 52.59,27.63 52.14,27.63 51.98,27.79 51.68,27.79 51.68,28.55 51.53,28.7 50.76,28.7 JP2.5
RX1  (via drill 0.2, 0.3)
  Top 0.152: 76.98,61.47 76.98,55.83 | IC1.45 66.62,61.76 v66.93,62.07
  Top 0.254: 86.73,91.19 86.73,99.11 86.43,99.42
  Top 0.305: v85.66,107.95 86.43,107.95 86.43,99.42 | 86.73,91.19 86.73,88.29 86.88,88.14 87.03,88.14 87.03,87.07 86.88,86.92 86.12,86.92 86.12,84.63 86.27,84.48 86.27,79.3 86.12,79.15 85.97,79.15 85.97,75.34 86.12,75.18 86.12,65.73 85.97,65.58 85.82,65.58 85.82,58.42 85.97,58.27 86.12,58.27 86.12,57.51 85.66,57.05 85.66,55.98 85.82,55.83 85.82,55.22 85.97,55.07 86.88,55.07 86.88,54 JP4.3 | v77.13,61.62 76.98,61.47 | 76.98,55.83 v77.13,55.68
  Bottom 0.152: v77.13,61.62 67.38,61.62 v66.93,62.07
  Bottom 0.305: v85.66,107.95 53.51,107.95 53.36,107.8 52.59,107.8 52.44,107.64 52.14,107.64 52.14,107.49 51.98,107.34 36.59,107.34 36.59,109.32 36.44,109.47 35.68,109.47 J3.1 | v77.13,55.68 77.28,55.83 84.9,55.83 85.05,55.68 85.05,54 86.73,54 JP4.3
RX_USB  (via drill 0.2)
  Top 0.305: v66.77,24.28 66.92,24.13 66.92,20.47 66.61,20.17 66.61,18.49 IC3.5 | v74.23,25.2 74.39,25.35 74.39,28.7 74.23,28.85 74.23,30.84 v74.08,30.99
  Bottom 0.305: v66.77,24.28 67.68,25.2 v74.23,25.2 | v74.08,30.99 73.93,31.14 68.59,31.14 68.44,30.99 65.39,30.99 65.09,31.29 63.41,31.29 JP2.16
SERR#  (via drill 0.2, 0.3)
  Top 0.152: X1.J3-A9 11.48,45.21 11.76,44.93 16.21,44.93 16.76,44.37 31.21,44.37 31.37,44.53 v31.69,44.53 | IC1.44 67.31,61.26 67.8,61.75 67.8,62.55 67.48,62.86 67.48,63.66 66.69,64.45 66.69,65.09 68.12,66.52 68.12,70.8 68.57,71.25 v68.57,71.99 68.44,72.12 68.44,74.45 69.04,75.06 v69.04,76.56
  Top 0.305: v80.48,71.68 80.33,71.83 80.33,72.75 80.18,72.75 80.03,72.9 80.03,79.15 82.16,79.15 82.31,79.3 82.31,80.21 R1.9 | v41.01,76.4 36.57,76.4 v36.53,76.36
  Bottom 0.152: v69.04,76.56 58.23,76.56 58.08,76.71 | 34.94,73.34 34.94,71.28 34.46,70.8 34.46,63.98 34.3,63.82 34.3,61.59 32.88,60.17 32.88,55.72 31.77,54.61 31.77,44.61 v31.69,44.53 | v68.57,71.99 68.84,71.99 68.91,71.91 80.25,71.91 v80.48,71.68
  Bottom 0.305: v80.48,71.68 80.33,71.83 | 58.08,76.71 41.47,76.71 41.31,76.56 41.16,76.56 v41.01,76.4 | v36.53,76.36 36.53,74.93 34.94,73.34
SRVBUS_0  (via drill 0.2, 0.3)
  Top 0.152: IC1.74 48.65,67.41 v47.96,68.1
  Top 0.305: v46.95,73.97 46.95,74.88 47.11,75.03 47.11,77.93 46.95,78.08 v46.95,90.42 | v64.33,90.27 64.17,90.42 64.17,98.04 64.33,98.2 64.33,99.87 64.17,100.03 63.11,100.03 63.11,109.02 v62.96,109.17
  Bottom 0.152: v47.96,68.1 47.96,69.37
  Bottom 0.305: v46.95,73.97 47.11,73.97 47.11,69.7 47.26,69.55 47.87,69.55 48.02,69.39 47.96,69.37 | v46.95,90.42 47.11,90.27 v64.33,90.27 | J8.1 63.32,109.54 arc90 v62.96,109.17
SRVBUS_1  (via drill 0.2, 0.3)
  Top 0.152: IC1.73 49.15,67.86 v48.91,68.1
  Top 0.305: J8.2 69.39,112.08 67.8,110.49 67.8,105.41 67.68,105.29 v67.68,105.23 | v48.17,73.97 48.17,74.88 48.02,75.03 48.02,77.93 48.17,78.08 48.17,78.84 48.02,78.99 47.41,78.99 47.41,89.97 47.56,90.12 v47.56,91.19 | v58.08,91.19 57.93,91.34 57.93,96.67 58.08,96.83 58.08,103.38 58.23,103.53 v58.23,105.24
  Bottom 0.152: v48.91,68.1 48.91,69.37
  Bottom 0.305: v48.17,73.97 47.56,73.97 47.56,70.16 47.72,70 48.17,70 48.48,69.7 48.48,69.55 48.63,69.55 48.78,69.39 48.94,69.39 48.91,69.37 | v47.56,91.19 47.72,91.34 57.93,91.34 v58.08,91.19 | v58.23,105.24 v67.67,105.24 v67.68,105.23
SRVBUS_2  (via drill 0.2, 0.3)
  Top 0.152: IC1.72 49.65,67.73 v49.86,67.94
  Top 0.305: J8.3 73.99,109.06 73.2,108.27 73.2,104.46 72.09,103.35 72.09,95.89 71.45,95.25 71.45,86.68 71.77,86.36 71.77,82.39 71.34,81.96 71.34,78.84 v71.49,78.69 | v49.09,73.97 v49.09,78.84
  Bottom 0.152: 49.55,69.37 49.86,69.06 v49.86,67.94
  Bottom 0.305: v49.09,73.97 48.94,73.97 48.94,72.75 49.09,72.59 49.55,72.59 49.55,69.37 | v49.09,78.84 49.24,78.69 57.47,78.69 57.62,78.84 71.34,78.84 v71.49,78.69
SRVBUS_3  (via drill 0.2, 0.3)
  Top 0.152: 73.04,110.65 | 72.88,110.49 73.04,110.65 | 72.88,110.49 | 72.72,110.33 72.88,110.49 | 71.14,95.89 70.66,95.41 70.66,85.09 | 71.62,104.47 71.61,104.46
  Top 0.305: J8.4 73.99,111.6 73.04,110.65 | v50.16,64.82 50.16,66.19 IC1.71 | v45.28,65.28 v45.28,68.17 | v45.73,73.97 v45.73,77.93 | 72.72,110.33 72.72,108.9 72.25,108.43 72.25,105.09 71.62,104.47 71.64,104.45 71.34,104.45 71.34,100.33 71.19,100.18 71.19,95.91 71.14,95.89 | v70.82,77.15 70.82,77.63 70.02,78.42 70.02,80.33 70.34,80.64 70.34,81.92 70.66,82.23 70.66,82.71 71.14,83.19 71.14,84.61 70.66,85.09
  Bottom 0.152: 45.89,77.78 58.08,77.78 58.23,77.93 58.84,77.93 59.76,77.01 68.3,77.01 68.44,77.15 | 68.44,77.15 | 68.44,77.15 68.59,77.31 70.66,77.31 v70.82,77.15
  Bottom 0.305: v50.16,64.82 50,64.67 47.41,64.67 46.95,65.13 45.43,65.13 v45.28,65.28 | v45.28,68.17 45.12,68.33 45.12,73.36 v45.73,73.97 | v45.73,77.93 45.89,77.78
SRVBUS_4  (via drill 0.2, 0.3)
  Top 0.152: IC1.19 57.15,46.05 58.28,44.93 58.28,44.61 58.75,44.13 58.75,43.34 59.07,43.02 v59.86,43.02
  Top 0.305: v76.98,86.46 76.83,86.31 76.83,71.37 v76.98,71.22 | v73.62,69.85 73.62,68.17 73.47,68.02 73.47,67.87 73.32,67.72 73.17,67.72 73.02,67.56 73.02,67.41 72.86,67.26 72.71,67.26 72.56,67.11 72.56,66.95 72.41,66.8 72.41,60.86 72.25,60.71 72.25,60.55 72.1,60.4 71.95,60.4 71.95,59.94 71.8,59.79 71.34,59.79 71.19,59.64 71.19,59.03 71.03,58.88 70.42,58.88 70.42,57.96 70.27,57.81 v69.97,57.81 | v69.81,55.37 70.12,55.37 70.12,55.07 70.42,54.76 71.19,54.76 v71.19,50.65 | J8.5 76.52,109.47 76.52,103.55 78.04,102.03 78.04,87.24 78.2,87.08 v78.51,86.77
  Bottom 0.152: v59.86,43.02 60.98,43.02 67.78,50.84
  Bottom 0.305: v76.98,71.22 77.13,71.07 77.59,71.07 77.74,70.92 77.74,69.7 76.83,69.7 76.67,69.85 v73.62,69.85 | v69.97,57.81 69.97,55.37 v69.81,55.37 | v71.19,50.65 71.03,50.8 67.83,50.8 67.78,50.84 | v76.98,86.46 78.2,86.46 v78.51,86.77
SRVBUS_5  (via drill 0.2, 0.3)
  Top 0.152: IC1.20 57.65,46.35 v59.55,44.45
  Top 0.305: v67.07,51.11 66.92,50.95 66.92,44.55 67.07,44.4 67.98,44.4 67.98,40.44 v68.14,40.28 | v98.77,37.08 98.62,37.24 98.62,40.74 98.77,40.89 99.38,40.89 99.38,41.05 99.53,41.2 99.53,42.27 99.38,42.42 99.23,42.42 99.23,46.23 99.38,46.38 99.38,46.53 99.53,46.69 99.69,46.69 99.84,46.84 100.75,46.84 100.9,46.69 101.82,46.69 101.82,52.78 101.67,52.93 99.38,52.93 99.38,55.37 99.23,55.52 98.77,55.52 98.77,82.65 99.08,82.96 99.08,87.63 99.39,87.95 99.39,88.27 98.92,88.74 98.92,88.9 98.44,89.38 98.44,89.83 v97.98,90.3 | v57.01,113.59 57.01,110.66 J1.3 | v79.87,91.03 78.91,91.99 78.75,102.55 77.64,103.66 77.8,110.17 77.01,110.97 77.01,111.6 J8.6
  Bottom 0.152: v59.55,44.45 61.13,44.45 66.93,51.09
  Bottom 0.305: v57.01,113.59 57.01,114.2 75.91,114.2 76.53,113.58 J8.6 | v67.07,51.11 66.92,51.11 66.93,51.09 | v68.14,40.28 77.59,40.28 77.74,40.13 77.74,39.22 79.42,39.22 79.57,39.06 79.57,36.02 85.21,36.02 85.36,35.86 85.36,35.1 98.16,35.1 98.31,35.25 98.31,37.08 v98.77,37.08 | v79.87,91.03 84.29,91.03 84.45,90.88 85.97,90.88 86.12,90.73 86.27,90.73 86.27,89.51 86.43,89.36 92.22,89.36 93.16,90.3 v97.98,90.3
SRVBUS_6  (via drill 0.2, 0.3)
  Top 0.152: IC1.21 58.15,46.64 58.75,46.04 59.23,45.56 v59.86,45.56
  Top 0.305: v71.8,59.18 71.95,59.03 73.47,59.03 v73.47,59.18 | v87.8,59.18 87.95,59.33 87.95,71.68 87.8,71.83 87.03,71.83 87.03,72.14 86.88,72.29 86.88,72.75 86.73,72.9 v86.73,74.42 | v80.33,81.74 80.18,81.89 80.18,84.18 80.33,84.33 80.64,84.33 80.64,92.86 80.48,93.02 80.33,93.02 80.33,103.84 80.18,103.99 79.11,103.99 79.11,109.47 J8.7 79.07,110.01 77.8,111.28 77.8,113.03 77.33,113.51 75.85,113.51 v75.45,113.11
  Bottom 0.152: v59.86,45.56 61.13,45.56 66.79,52 66.85,52.07
  Bottom 0.305: J1.4 55.95,112.06 56.68,112.06 58.06,113.45 | v71.8,59.18 66.77,59.18 66.77,52.02 66.79,52 | v73.47,59.18 75.3,59.18 75.45,59.03 87.64,59.03 v87.8,59.18 | v86.73,74.42 84.6,74.42 84.45,74.57 84.45,81.74 v80.33,81.74 | 58.06,113.45 58.12,113.51 | v75.45,113.11 75.18,113.11 74.79,113.51 58.16,113.51 58.08,113.44 58.06,113.45
SRVBUS_7  (via drill 0.2, 0.3)
  Top 0.152: IC1.22 58.65,47.09 v59.23,46.51
  Top 0.305: v65.24,51.11 65.39,51.26 66.46,51.26 66.46,46.08 66.31,45.92 66.31,42.57 66.46,42.42 v66.77,42.42 | v95.42,43.18 95.42,44.09 95.57,44.25 95.57,46.84 95.42,46.99 95.42,50.8 95.57,50.95 v96.64,50.95 | v98.31,87.83 98.31,85.24 98.47,85.09 98.47,83.11 98.31,82.96 98.31,58.7 v98.02,58.41 | J8.8 79.11,112.22 79.11,114.35 83.68,114.35 83.83,114.2 83.83,111 83.99,110.85 83.99,103.67 85.26,102.39 | 85.26,102.39 | 85.26,102.39 85.42,102.23 85.42,90.81 85.58,90.65 | 85.58,90.65 | 85.58,90.65 86.06,90.17 86.06,87.9 v86.27,87.68
  Bottom 0.152: v59.23,46.51 60.82,46.51 64.92,51.12
  Bottom 0.305: v65.24,51.11 64.94,51.11 64.92,51.12 | v66.77,42.42 75.61,42.42 75.76,42.57 75.76,43.33 78.65,43.33 78.81,43.48 78.96,43.48 79.11,43.64 89.02,43.64 89.17,43.48 89.17,43.33 95.27,43.33 v95.42,43.18 | v96.64,50.95 96.79,51.11 99.08,51.11 99.23,51.26 99.23,51.71 99.38,51.87 99.38,55.37 98.31,56.44 98.31,57.95 98.02,58.24 v98.02,58.41 | v98.31,87.83 98.16,87.68 93.59,87.68 93.44,87.53 86.43,87.53 v86.27,87.68 | J1.1 54.62,110.81 78.44,110.81 79.07,111.44 J8.8
SSW1#  (via drill 0.2)
  Top 0.152: 62.35,74.12 62.35,70.92 62.5,70.76 62.5,70.16 62.65,70 | 62.5,65.13 62.46,65.09 61.61,65.09 61.21,64.69 56.53,64.69 56.15,65.07 IC1.59
  Top 0.305: v62.35,91.8 62.5,91.64 62.5,89.05 62.35,88.9 62.35,86.61 62.04,86.31 62.04,79.91 62.35,79.6 62.35,78.69 62.04,78.38 62.04,74.42 62.35,74.12 | 62.65,70 62.65,65.28 62.5,65.13 | v78.2,25.65 78.04,25.81 78.04,28.85 v78.2,29.01 | v106.54,27.94 106.7,28.09 106.7,43.94 106.54,44.09 105.17,44.09 105.17,46.23 105.32,46.38 105.32,46.69 105.48,46.84 106.08,46.84 106.08,62.23 105.78,62.53 105.78,63.14 106.24,63.6 106.7,63.6 106.7,94.39 v106.54,94.54 | v20.13,7.67 20.59,8.13 20.59,14.99 v20.44,15.14 | v25.92,15.14 v25.92,23.22
  Bottom 0.254: 86.53,92.71 94.35,92.71 94.81,93.17
  Bottom 0.305: v62.35,91.8 66.61,91.8 66.77,91.64 67.38,91.64 67.53,91.8 73.4,91.8 R6.1 | v78.2,25.65 78.04,25.81 73.47,25.81 73.32,25.65 63.87,25.65 63.87,23.98 63.72,23.82 44.97,23.82 44.21,23.06 26.07,23.06 v25.92,23.22 | v78.2,29.01 86.43,29.01 86.73,29.31 92.83,29.31 92.98,29.16 92.98,28.55 95.72,28.55 95.88,28.4 95.88,27.63 106.08,27.63 106.24,27.79 106.39,27.79 v106.54,27.94 | v106.54,94.54 94.96,94.54 94.81,94.39 94.81,93.17 | R6.1 82.09,92.55 83.52,93.98 84.95,93.98 86.22,92.71 86.53,92.71 | R6.1 | v20.13,7.67 16.93,7.67 JP12.2 | v20.44,15.14 v25.92,15.14
SSW2#  (via drill 0.2, 0.3, 0.6)
  Top 0.152: R7.1 74.15,80.49 75.1,79.53 75.1,77.31 73.99,76.2 73.99,73.98 v73.52,73.5 | v61.79,68.54 61.93,68.74 61.93,73.03 v61.61,73.34 | IC1.60 55.65,67.4 55.64,68.92 55.78,69.25 | 53.36,1.59 57.32,1.59 57.96,2.22 | 57.96,2.22 | v55.84,69.25 55.78,69.25 | 55.78,69.25
  Top 0.305: v104.71,86 104.87,85.85 104.87,64.52 104.71,64.36 104.1,64.36 104.1,63.75 103.95,63.6 v103.95,60.25 | v104.1,56.29 104.26,56.13 104.26,49.43 104.1,49.28 103.95,49.28 103.95,47.75 104.1,47.6 104.1,46.69 103.95,46.53 103.95,45.62 103.8,45.47 101.82,45.47 101.82,45.01 101.67,44.86 101.67,43.94 101.82,43.79 101.82,42.27 101.67,42.11 101.67,41.2 101.82,41.05 v101.82,37.85 | v85.36,37.69 85.36,33.12 85.51,32.97 85.82,32.97 85.82,27.33 85.66,27.18 v85.66,23.67 | v79.87,9.96 v79.87,23.52
  Top 0.406: JP13.2 13.03,7.62 14.14,6.51 14.14,3.33 15.89,1.59 53.36,1.59 | 57.96,2.22 57.96,8.89 v59.39,10.32
  Bottom 0.152: v73.52,73.5 71.61,73.5 71.14,73.98 69.86,73.98 69.55,73.66 68.44,73.66 67.64,74.45 62.56,74.45 61.61,73.5 v61.61,73.34 | 59.23,68.42 58.44,69.22 55.88,69.22 v55.84,69.25 | 59.23,68.42 | 59.23,68.42 59.39,68.26 61.51,68.26 v61.79,68.54
  Bottom 0.305: v104.71,86 104.56,86.16 94.35,86.16 94.2,86 82.92,86 82.92,84.33 82.77,84.18 74.23,84.18 R7.1 | v103.95,60.25 104.1,60.1 104.71,60.1 104.87,59.94 104.87,56.44 104.56,56.44 104.41,56.29 v104.1,56.29 | v101.82,37.85 92.98,37.85 92.83,37.69 92.22,37.69 92.06,37.85 87.03,37.85 86.88,37.69 v85.36,37.69 | v85.66,23.67 85.51,23.52 81.09,23.52 80.94,23.67 80.03,23.67 v79.87,23.52 | v79.87,9.96 79.72,10.11
  Bottom 0.406: v59.39,10.32 64.31,10.32 64.94,9.68 77.8,9.68 78.44,10.32 79.51,10.32 v79.87,9.96
STOP#  (via drill 0.2, 0.3)
  Top 0.152: X1.J3-A11 13.19,49.21 14.3,48.1 15.41,48.1 16.68,46.83 17.08,46.83 17.8,46.12 28.51,46.12 v28.83,46.43 | IC1.56 57.65,67.3 57.64,67.31 57.8,67.47 57.8,67.79 57.96,67.94 | 60.02,86.01 60.02,80.64 60.18,80.49 60.18,74.45 | 58.12,71.6 58.12,68.1 57.96,67.94 | 57.96,67.94
  Top 0.254: v57.88,72.87 57.88,72.47 58.12,72.23 58.12,71.6
  Top 0.305: v79.26,70.16 79.11,70.31 79.11,72.29 78.81,72.59 78.81,79.45 79.11,79.76 79.11,84.63 79.26,84.78 v79.26,86.16 | 32.78,76.56 v32.72,76.52 33.19,76.99 33.19,82.07 33.51,82.39 34.46,82.39 36.13,84.06 v36.13,86.77 | 60.02,86.01 60.12,86.11 v60.12,86.68 | v59.35,72.69 60.18,73.52 60.18,74.45
  Bottom 0.152: v32.72,76.52 32.72,75.25 32.72,64.93 32.24,64.45 32.24,62.39 30.81,60.96 | 60.18,86.68 v60.12,86.68 60.02,86.68 | 59.86,85.85 60.02,86.01 | v28.83,46.43 28.83,47.55 29.23,47.94 29.23,55.09 30.81,56.67 | v57.88,72.87 59.17,72.87 v59.35,72.69
  Bottom 0.305: v79.26,70.16 82.16,70.16 R1.5 | v79.26,86.16 79.11,86 77.59,86 77.43,85.85 59.86,85.85 55.95,85.85 55.79,86 55.79,86.77 54.57,86.77 54.42,86.61 54.42,86.46 39.49,86.46 39.33,86.61 37.35,86.61 37.2,86.77 v36.13,86.77 | 30.81,56.67 30.81,60.96 | v60.12,86.68 60.06,86.61 60.06,86 60.02,86.01
TRDY#  (via drill 0.2, 0.3)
